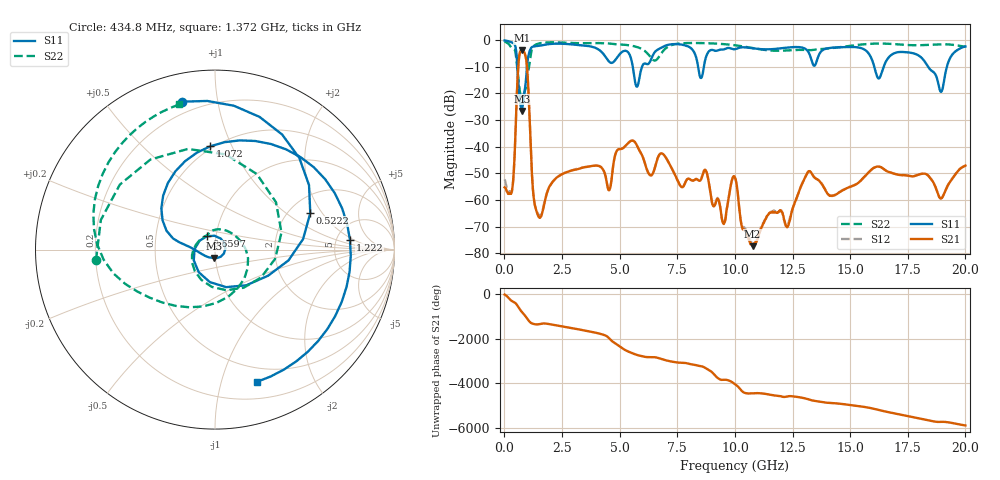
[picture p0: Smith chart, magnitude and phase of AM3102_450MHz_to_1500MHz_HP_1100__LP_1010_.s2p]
!Agilent Technologies,E8364B,MY43040894,A.07.50.67
!Agilent E8364B: A.07.50.67
!Date: Thursday, January 11, 2018 06:34:45
!Correction: S11(Full 2 Port(1,2))
!S21(Full 2 Port(1,2))
!S12(Full 2 Port(1,2))
!S22(Full 2 Port(1,2))
!S2P File: Measurements: S11, S21, S12, S22:
# Hz S  dB  R 50
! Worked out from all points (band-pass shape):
!   1601 points, 10 MHz to 20 GHz, reference 50 ohm
!   highest |S21| = -3.71 dB at 759.6 MHz (marker M1); lowest = -77.4 dB at 10.77 GHz (marker M2)
!   |S21| within 3 dB of the highest: 634.6 MHz to 934.9 MHz (300.3 MHz wide, 38.3 % of centre)
!   lowest |S11| = -26.6 dB at 759.6 MHz (marker M3), VSWR 1.10, Z = 49.1 - j4.56 ohm
!   |S11| at or under -10 dB: 562.1 MHz to 979.6 MHz (417.5 MHz wide, 54.2 % of centre); 16.05 GHz to 16.45 GHz (402.7 MHz wide, 2.48 % of centre); 18.38 GHz to 19.2 GHz (812.9 MHz wide, 4.33 % of centre)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
!   |S22| runs from -21.0 to -0.5 dB; largest |S21 - S12| = 0.00095
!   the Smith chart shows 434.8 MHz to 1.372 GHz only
!   S11 on the Smith chart (normalised r, x): 434.8 MHz: 0.14, +0.79; 522.2 MHz: 2.59, +1.56; 659.7 MHz: 0.91, +0.14; 1.072 GHz: 0.48, +0.83; 1.222 GHz: 6.69, +1.70; 1.372 GHz: 0.36, -1.30
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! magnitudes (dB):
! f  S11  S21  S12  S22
! 10 MHz  -0.1  -55.3  -52.2  -0.5
! 284.9 MHz  -0.7  -57.4  -57.1  -2.6
! 434.8 MHz  -1.5  -45.0  -45.1  -3.5
! 522.2 MHz  -4.9  -24.5  -24.5  -7.3
! 659.7 MHz  -21.2  -5.1  -5.1  -18.5
! 759.6 MHz  -26.6  -3.7  -3.7  -20.9
! 1.072 GHz  -4.8  -24.5  -24.5  -9.8
! 1.222 GHz  -2.5  -54.1  -54.1  -2.8
! 1.372 GHz  -2.2  -63.6  -63.4  -1.6
! 3.346 GHz  -1.9  -48.0  -47.9  -1.1
! 4.545 GHz  -8.1  -56.4  -56.3  -1.2
! 5.332 GHz  -4.3  -38.9  -38.9  -1.8
! 5.745 GHz  -17.5  -39.4  -39.4  -2.5
! 6.682 GHz  -3.4  -43.7  -43.6  -6.5
! 8.731 GHz  -6.8  -48.8  -48.8  -1.1
! 9.505 GHz  -3.5  -68.9  -69.0  -1.4
! 10.01 GHz  -3.4  -51.6  -51.6  -1.9
! 10.77 GHz  -3.0  -77.4  -76.8  -2.9
! 13.34 GHz  -8.0  -50.1  -50.1  -3.7
! 16.68 GHz  -6.4  -49.5  -49.5  -1.3
! 18.94 GHz  -19.4  -59.5  -59.3  -1.5
! 20 GHz  -2.3  -47.1  -47.2  -2.4
